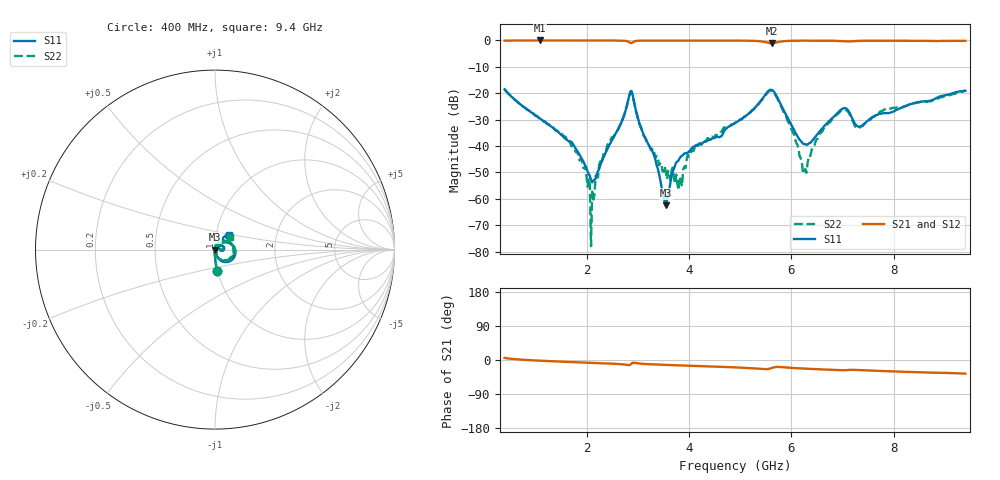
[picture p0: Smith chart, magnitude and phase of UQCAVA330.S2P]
!  Part Number  UQCAVA330 Mounting Orientation: Horizontal
!  Description: RF capacitors
!  Application: Coupling, Bypass, Tuning, DC Block
!  Filters, Matching
# GHZ S DB R 50
! Freq  |S11|  S11 Ph  |S21|  S21 Ph  |S12|  S12 Ph  |S22|  S22 Ph
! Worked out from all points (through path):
!   401 points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, 400 MHz to 9.4 GHz, reference 50 ohm
!   highest |S21| = -0.02 dB at 1.098 GHz (marker M1); lowest = -1.1 dB at 5.62 GHz (marker M2)
!   group delay of S21, straight-line fit = 11.2 ps
!   lowest |S11| = -62.5 dB at 3.55 GHz (marker M3), VSWR 1.00, Z = 49.9 + j0.0386 ohm
!   |S11| at or under -10 dB: start of sweep to end of sweep
!   |S22| runs from -77.9 to -18.5 dB; largest |S21 - S12| = 0.0035
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0.4  -18.55 -84.3  -0.07 5.4  -0.06 5.4  -18.51 -83.9
1.098  -29.65 -90.2  -0.02 -1.9  -0.01 -2.0  -29.68 -88.8
1.908  -44.90 -77.6  -0.03 -6.4  -0.02 -6.4  -45.13 -91.1
2.11  -53.77 -17.2  -0.03 -7.4  -0.03 -7.5  -57.24 18.9
2.29  -46.14 53.7  -0.04 -8.4  -0.03 -8.4  -46.63 71.3
2.875  -19.14 -15.8  -1.04 -9.7  -1.03 -9.8  -19.34 -13.7
3.145  -36.86 -88.9  -0.08 -10.6  -0.07 -10.6  -36.66 -72.8
3.415  -50.42 -123.2  -0.05 -12.2  -0.04 -12.3  -47.29 -52.9
3.55  -62.51 149.0  -0.05 -12.9  -0.05 -13.0  -49.96 -37.0
3.708  -48.62 101.5  -0.06 -13.7  -0.05 -13.8  -52.28 -11.4
3.82  -44.56 86.2  -0.06 -14.2  -0.05 -14.3  -51.63 54.8
3.865  -43.69 79.9  -0.06 -14.4  -0.05 -14.5  -55.27 94.4
4.158  -39.56 66.1  -0.06 -15.7  -0.05 -15.8  -39.96 81.8
4.9  -31.29 57.2  -0.08 -19.4  -0.07 -19.5  -31.21 71.0
5.62  -18.74 -21.2  -1.10 -21.0  -1.10 -21.1  -19.09 -14.2
6.003  -32.11 -71.6  -0.15 -20.8  -0.15 -20.9  -33.73 -82.2
6.25  -39.29 -27.2  -0.10 -22.6  -0.10 -22.8  -50.03 -10.1
6.408  -37.98 14.7  -0.09 -23.6  -0.09 -23.7  -40.62 54.7
6.993  -25.98 20.4  -0.30 -27.1  -0.31 -27.2  -26.48 33.2
7.308  -32.67 10.7  -0.18 -26.4  -0.18 -26.6  -33.26 21.5
7.915  -27.46 43.9  -0.09 -29.8  -0.10 -29.9  -25.78 43.8
9.4  -19.10 47.1  -0.16 -35.9  -0.18 -36.0  -19.02 39.9
